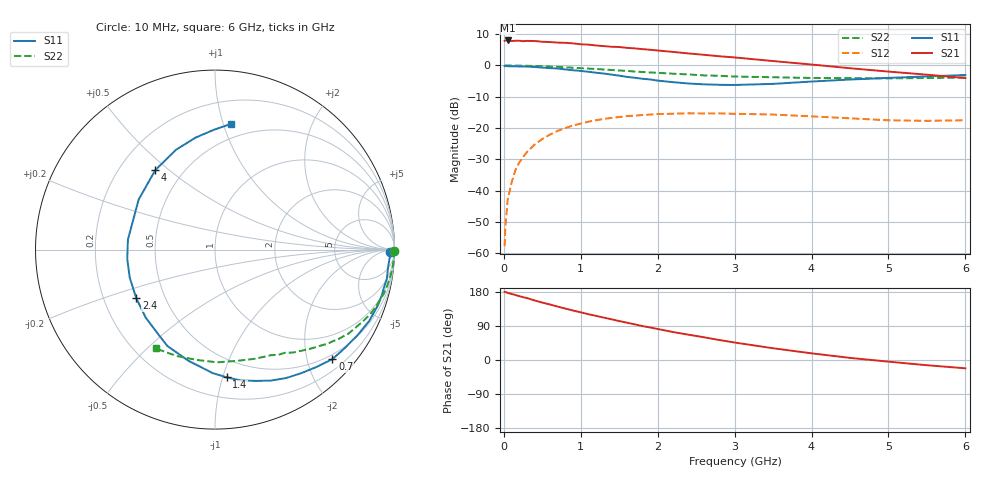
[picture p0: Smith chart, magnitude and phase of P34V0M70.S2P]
! SIEMENS Small Signal Semiconductors
! BFP181
! Si NPN RF Bipolar Junction Transistor in SOT143
! VCE = 4 V  IC = 0.7 mA
! Common Emitter S-Parameters:  March  1996
# GHz  S  MA  R  50
!  f  S11  S21  S12  S22
! GHz  MAG  ANG  MAG  ANG  MAG  ANG  MAG  ANG
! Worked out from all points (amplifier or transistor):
!   36 points, 10 MHz to 6 GHz, reference 50 ohm
!   highest |S21| = 8.0 dB at 50 MHz (marker M1)
!   |S21| within 3 dB of that: start of sweep to 1.913 GHz
!   unconditionally stable (mu >= 1): 3.524 GHz to end of sweep
!   at 250 MHz: K = 0.08, MSG = 18.5 dB, |S12| = -29.3 dB
!   at 1.4 GHz: K = 0.44, MSG = 11.4 dB, |S12| = -16.7 dB
!   at 6 GHz: K = 1.36, MAG = 3.2 dB, |S12| = -17.5 dB
!   S11 on the Smith chart (normalised r, x): 10 MHz: 63, -30; 700 MHz: 0.41, -2.48; 1.4 GHz: 0.35, -1.03; 2.4 GHz: 0.34, -0.25; 4 GHz: 0.35, +0.45; 6 GHz: 0.38, +1.06
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0.01  0.9746 -0.7  2.476 179.8  0.0013 78.2  0.999 -0.3
0.02  0.983 -1.1  2.509 179.5  0.0027 81.7  0.9981 -0.5
0.05  0.974 -2.8  2.511 177.2  0.0072 90.1  0.9981 -1.5
0.1  0.9692 -6.2  2.453 174.4  0.0134 84.2  0.997 -3.0
0.15  0.9715 -9.6  2.485 171.5  0.0212 82.5  0.9952 -4.4
0.25  0.9635 -15.3  2.446 165.8  0.0344 79.7  0.991 -7.4
0.3  0.9597 -18.7  2.469 163.5  0.0413 77.1  0.9877 -8.8
0.4  0.9467 -24.8  2.462 157.1  0.0545 73.1  0.9809 -11.7
0.7  0.8946 -43.0  2.32 140.9  0.0902 60.6  0.9491 -20.0
0.9  0.8399 -55.0  2.256 130.6  0.1101 52.8  0.9206 -25.1
1.1  0.7932 -67.0  2.154 120.8  0.1266 45.8  0.892 -29.7
1.4  0.7148 -84.7  1.992 107.4  0.1455 36.1  0.8477 -36.2
1.5  0.6882 -91.1  1.973 102.7  0.1504 33.3  0.831 -37.9
1.7  0.6373 -103.3  1.878 94.1  0.1583 28.1  0.8005 -41.7
2.2  0.5411 -135.5  1.646 73.8  0.1698 16.3  0.7389 -49.8
2.4  0.5157 -148.2  1.558 66.8  0.1723 12.0  0.7194 -52.9
3  0.4884 173.5  1.345 46.1  0.1691 2.0  0.6665 -61.9
3.5  0.5087 146.7  1.177 31.0  0.1646 -4.3  0.6487 -69.5
4  0.5539 126.9  1.036 17.6  0.154 -8.6  0.6322 -78.6
4.5  0.5972 111.3  0.904 5.6  0.1433 -11.3  0.6282 -88.8
5.5  0.6681 90.4  0.713 -13.8  0.1307 -7.1  0.6303 -109.9
6  0.705 82.9  0.63 -21.9  0.1334 -4.4  0.6421 -120.9
